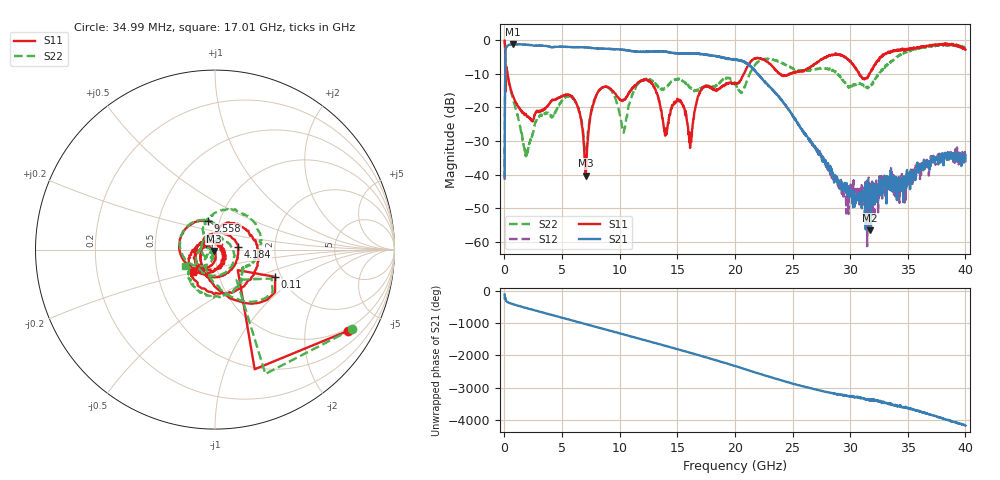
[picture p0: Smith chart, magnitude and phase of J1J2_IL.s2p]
!Agilent Technologies,N5230A,US43500312,A.07.50.67
!Agilent N5230A: A.07.50.67
!Date: Thursday, March 05, 2015 11:13:44
!Correction: S11(Full 2 Port(1,2))
!S21(Full 2 Port(1,2))
!S12(Full 2 Port(1,2))
!S22(Full 2 Port(1,2))
!S2P File: Measurements: S11, S21, S12, S22:
# Hz S  dB  R 50
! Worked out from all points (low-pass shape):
!   1601 points, 10 MHz to 40 GHz, reference 50 ohm
!   highest |S21| = -1.15 dB at 759.8 MHz (marker M1); lowest = -56.7 dB at 31.73 GHz (marker M2)
!   |S21| within 3 dB of the highest: 81.97 MHz to 17.15 GHz (17.07 GHz wide, 198 % of centre); 17.21217 GHz to 17.26001 GHz (47.85 MHz wide, 0.278 % of centre)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
!   lowest |S11| = -40.3 dB at 7.058 GHz (marker M3), VSWR 1.02, Z = 49.4 - j0.734 ohm
!   |S11| at or under -10 dB: 261.1 MHz to 20.78 GHz (20.52 GHz wide, 195 % of centre); 23.9 GHz to 24.7 GHz (802.3 MHz wide, 3.3 % of centre); 30.77 GHz to 31.68 GHz (909.4 MHz wide, 2.91 % of centre)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
!   |S22| runs from -35.0 to -0.1 dB; largest |S21 - S12| = 0.015
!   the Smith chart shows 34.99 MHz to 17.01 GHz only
!   S11 on the Smith chart (normalised r, x): 34.99 MHz: 0.90, -3.34; 110 MHz: 1.86, -0.65; 4.184 GHz: 1.29, +0.04; 9.558 GHz: 0.88, +0.29; 17.01 GHz: 0.76, -0.19
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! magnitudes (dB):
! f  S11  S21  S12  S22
! 10 MHz  -0.1  -40.6  -41.6  -0.1
! 34.99 MHz  -1.2  -19.1  -19.1  -1.1
! 110 MHz  -8.7  -2.4  -2.3  -9.0
! 284.9 MHz  -10.5  -1.6  -1.6  -10.7
! 759.8 MHz  -16.7  -1.2  -1.2  -17.7
! 1.885 GHz  -22.4  -1.3  -1.3  -33.6
! 4.184 GHz  -17.8  -2.1  -2.1  -22.8
! 6.683 GHz  -24.6  -2.1  -2.1  -23.7
! 7.058 GHz  -40.3  -2.1  -2.1  -35.0
! 8.008 GHz  -16.2  -2.5  -2.4  -16.0
! 9.558 GHz  -15.7  -2.7  -2.6  -16.7
! 10.33 GHz  -17.8  -2.8  -2.9  -27.5
! 11.63 GHz  -12.6  -3.4  -3.4  -12.9
! 13.36 GHz  -17.4  -3.2  -3.3  -13.8
! 16.11 GHz  -32.1  -3.8  -3.9  -14.1
! 17.01 GHz  -15.1  -4.1  -4.1  -14.4
! 20 GHz  -12.9  -5.8  -5.8  -12.8
! 26.68 GHz  -7.7  -30.5  -31.0  -8.9
! 29.7 GHz  -5.5  -42.6  -44.5  -13.4
! 31.73 GHz  -9.7  -56.7  -42.8  -13.7
! 33.35 GHz  -3.5  -43.7  -42.4  -7.0
! 40 GHz  -2.8  -36.0  -34.2  -1.9
